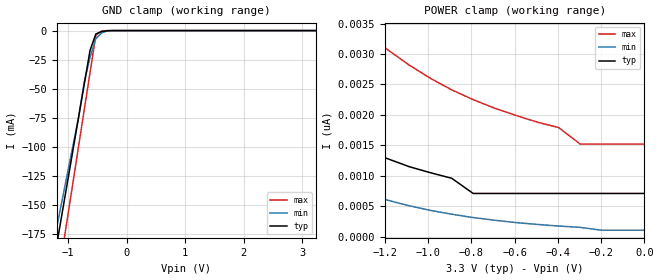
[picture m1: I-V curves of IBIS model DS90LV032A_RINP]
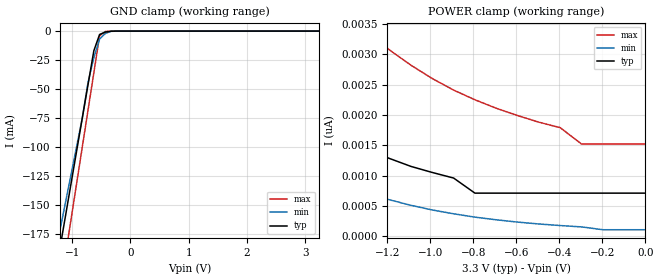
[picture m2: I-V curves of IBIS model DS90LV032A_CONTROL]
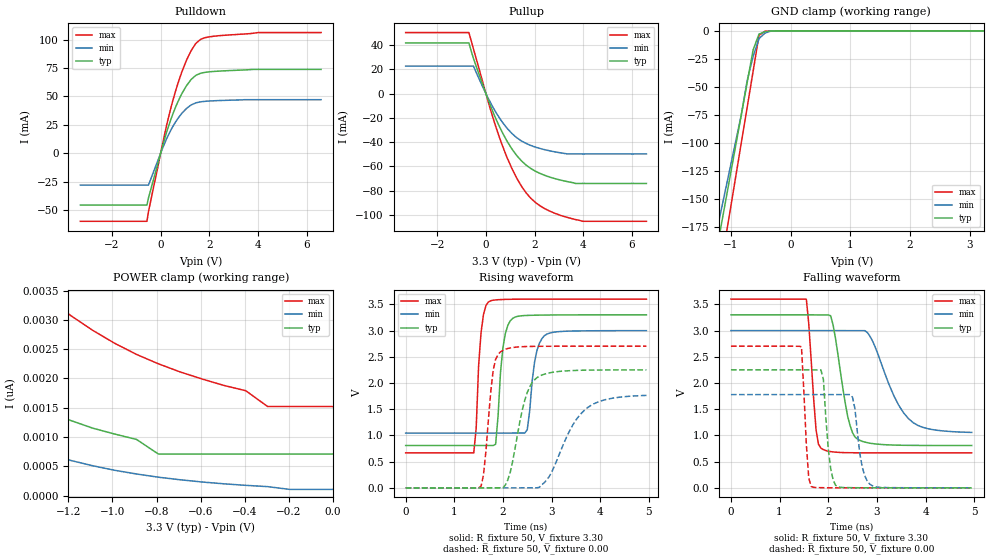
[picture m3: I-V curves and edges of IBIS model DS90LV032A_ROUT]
|   National Semiconductor Corporation
|   IBIS Model of DS90LV032A
|   3V LVDS Quad CMOS Differential Line Receiver
|   16 Lead SOIC Package
[IBIS Ver]   3.2
[Comment Char]   |_char
[File name]   ds90lv032atm.ibs
[File Rev]   2.2
[Date]   01/21/04
[Source]   SPICE to IBIS Translation
[Notes]
IBIS Parser Results:
Checking ds90lv032atm.ibs for IBIS 3.2 Compatibility...
Errors  : 0
File Passed
* Rev 2.2 Comments:
- Revision date: 01/21/04
Model Comments:
- Corrected [Difff Pin] assignments for pin 14 and 15
- Modifed [Diff Pin} comments
Modified By: DG
* END Rev 2.2 Comments
* Rev 2.1 Comments:
- Revision date: 06/03/03
Model Comments:
- Updated package parasitics data- added min/max
- Modifed fall and rise waveforms so that they are monotonic
- Corrected gnd clamp and power clamp data
Modified By: DG
* END Rev 2.1 Comments
* Rev 1.1 Comments:
- Revision date: 03/20/03
Model Comments:
- This file includes typ/min/max data
- SPICE files used were from an equivalent I/O design cell
- The CONTROL Model represents the following pins: EN, ENb
Created By: Tim Coyle
* END Rev 1.1 Comments
[Disclaimer]
(C) Copyright National Semiconductor Corporation 2003
   All rights reserved
   National Semiconductor Corporation hereby grants
the user of this IBIS model a non-exclusive, nontransferable
license to use this IBIS model under the following terms.
Before using this IBIS model, the user should read this
license.  If the user does not accept these terms,  the
IBIS model should be returned to National within 30 days.
   The user is granted this license only to use the
IBIS model and is not granted rights to sell, load, rent,
lease or license the IBIS model in whole or in part, or in
modified form to anyone other than user. User may modify
the IBIS model to suit its specific applications but rights
to derivative works and such modifications shall belong to
National.
   This IBIS model is provided on an "AS IS" basis and
National makes absolutely no warranty with respect to the
information contained herein.NATIONAL DISCLAIMS AND CUSTOMER
WAIVES ALL WARRANTIES, EXPRESS OR IMPLIED, INCLUDING
WARRANTIES OF MERCHANTABILITY OR FITNESS FOR A PARTICULAR
PURPOSE. The entire risk as to quality and performance is
with the Customer. ACCORDINGLY, IN NO EVENT SHALL THE
COMPANY BE LIABLE FOR ANY DAMAGES, WHETHER IN CONTRACT OR
TORT,INCLUDING ANY LOST PROFITS OR OTHER INCIDENTAL,
CONSEQUENTIAL, EXEMPLARY, OR PUNITIVE DAMAGES ARISING OUT
OF THE USE OR APPLICATION OF THE IBIS model provided in
this package.Further, National reserves the right to make
changes without notice to any product herein to improve
reliability, function, or design. National does not convey
any license under patent rights or any other intellectual
property rights, including those of third parties.
   National is not obligated to provide maintenance or support
for the licensed IBIS model.
Contact National at
   ATTN:INTERFACE APPLICATIONS/IBIS MODELS
   5 Foden Road, M/S 03-03
   South Porltand, ME 04106
   (207) 541-6031
[Copyright]   (c) Copyright 2003 National Semiconductor Corp.
[Component]   DS90LV032ATM
Si_location Pin
Timing_location Pin
[Manufacturer]   National Semiconductor Corp.
[Package]
|   TYP   MIN   MAX
R_pkg   50.0m   50.0m   50.0m
L_pkg   1.37nH  0.95n   2.07n
C_pkg   0.26pF  0.146p  0.429p
[Pin]   signal_name   model_name   R_pin   L_pin   C_pin
1   Rin1-   DS90LV032A_RINM   50.0m   2.07n   0.429p
2   Rin1+   DS90LV032A_RINP   50.0m   1.49n   0.306p
3   Rout1   DS90LV032A_ROUT   50.0m   0.95n   0.146p
4   EN   DS90LV032A_CONTROL 50.0m   0.95n   0.152p
5   Rout2   DS90LV032A_ROUT   50.0m   0.95n   0.152p
6   Rin2+   DS90LV032A_RINP   50.0m   0.95n   0.146p
7   Rin2-   DS90LV032A_RINM   50.0m   1.49n   0.306p
8   GND   GND   50.0m   2.07n   0.429p
9   Rin3-   DS90LV032A_RINM   50.0m   2.07n   0.429p
10   Rin3+   DS90LV032A_RINP   50.0m   1.49n   0.306p
11   Rout3   DS90LV032A_ROUT   50.0m   0.95n   0.146p
12   EN*   DS90LV032A_CONTROL 50.0m   0.95n   0.152p
13   Rout4   DS90LV032A_ROUT   50.0m   0.95n   0.152p
14   Rin4+   DS90LV032A_RINP   50.0m   0.95n   0.146p
15   Rin4-   DS90LV032A_RINM   50.0m   1.49n   0.306p
16   Vcc   POWER   50.0m   2.07n   0.429p
[Diff Pin] inv_pin   vdiff   tdelay_typ   tdelay_min   tdelay_max
| The '+' pin is Diff_pin and the '-' pin is the inv_pin
| Vdiff for Inputs is differential threshold Vth/Vtl (from datasheet)
| Vdiff is 0 for Outputs
| The 'tdelay' parameters are for specifying launch delays of the
| non-inverting pin relative to the inverting pin
| The 'tdelay' for Inputs is NA;  For LVDS Outputs it is 0ns since there
| is no transistor delay between the diff. pairs;
| the package delay is reflected by the  L_pin in the [Pin] keyword.
2   1   100mV   NA   NA   NA
6   7   100mV   NA   NA   NA
10   9   100mV   NA   NA   NA
14   15   100mV   NA   NA   NA
| Models and submodels in the file (4): DS90LV032A_RINP (Input), DS90LV032A_RINM (Input), DS90LV032A_CONTROL (Input), DS90LV032A_ROUT (3-state)
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[Model]   DS90LV032A_RINP
Model_type Input
Vinh=0.1
Vinl=-0.1
|   TYP   MIN   MAX
C_comp   2.25p   1p   2.75p
[Temperature Range] 25   85   -40
[Voltage Range]   3.30   3.00   3.60
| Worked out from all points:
|   GND clamp passes 1 mA (typ) near -0.44 V on its own axis
[GND Clamp]
|V(groundclamp)   I(typ)   I(min)   I(max)
-3.3V     -800mA     -700mA     -900mA
-1.221V   -191mA     -175mA     -228mA
-1.122V   -162mA     -150mA     -196mA
-1.023V   -133mA     -125mA     -164mA
-825mV    -75mA      -75mA      -100mA
-726mV    -46mA      -44.2mA    -68mA
-627mV    -17mA      -22.9mA    -36mA
-528mV    -2.88mA    -6.91mA    -4mA
-429mV    -868uA     -2.06mA    -342uA
-330mV    -103uA     -230uA     -43.7uA
-231mV    -7.76uA    -11.5uA    -4.83uA
3.234V    245pA      53.3pA     1.12nA
[POWER Clamp]
|V(table)   I(typ)   I(min)   I(max)
-3.267V   19.9nA     16nA       32nA
-2.277V   5.16nA     3.62nA     10.2nA
-2.178V   4.5nA      3.09nA     9.04nA
-1.98V    3.42nA     2.24nA     7.15nA
-1.683V   2.29nA     1.37nA     5.09nA
-1.287V   1.42nA     707pA      3.37nA
-1.089V   1.15nA     508pA      2.82nA
-891mV    958pA      368pA      2.41nA
-792mV    709pA      313pA      2.25nA
-396mV    709pA      174pA      1.79nA
-297mV    709pA      152pA      1.52nA
0V        709pA      105pA      1.52nA
[Model]   DS90LV032A_CONTROL
Model_type Input
Vinh=2.0
Vinl=0.8
|   TYP   MIN   MAX
C_comp   3p   3p   3p
[Temperature Range] 25   85   -40
[Voltage Range]   3.30   3.00   3.60
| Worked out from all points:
|   GND clamp passes 1 mA (typ) near -0.44 V on its own axis
[GND Clamp]
|V(groundclamp)   I(typ)   I(min)   I(max)
-3.3V     -800mA     -700mA     -900mA
-1.221V   -191mA     -175mA     -228mA
-1.122V   -162mA     -150mA     -196mA
-1.023V   -133mA     -125mA     -164mA
-825mV    -75mA      -75mA      -100mA
-726mV    -46mA      -44.2mA    -68mA
-627mV    -17mA      -22.9mA    -36mA
-528mV    -2.88mA    -6.91mA    -4mA
-429mV    -868uA     -2.06mA    -342uA
-330mV    -103uA     -230uA     -43.7uA
-231mV    -7.76uA    -11.5uA    -4.83uA
3.234V    245pA      53.3pA     1.12nA
[POWER Clamp]
|V(table)   I(typ)   I(min)   I(max)
-3.267V   19.9nA     16nA       32nA
-2.277V   5.16nA     3.62nA     10.2nA
-2.178V   4.5nA      3.09nA     9.04nA
-1.98V    3.42nA     2.24nA     7.15nA
-1.683V   2.29nA     1.37nA     5.09nA
-1.287V   1.42nA     707pA      3.37nA
-1.089V   1.15nA     508pA      2.82nA
-891mV    958pA      368pA      2.41nA
-792mV    709pA      313pA      2.25nA
-396mV    709pA      174pA      1.79nA
-297mV    709pA      152pA      1.52nA
0V        709pA      105pA      1.52nA
[Model]   DS90LV032A_ROUT
Model_type 3-state
Enable Active-High
Polarity Non-Inverting
Vref=0.0
Vmeas=1.65
Cref=10p
|   TYP   MIN   MAX
C_comp   4.2p   3.7p   4.9p
[Temperature Range] 25   85   -40
[Voltage Range]   3.30   3.00   3.60
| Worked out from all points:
|   slope of the pulldown table from 0 to 0.495 V, typ, clamps not added: 14.5 ohm
|   slope of the pullup table from 0 to 0.495 V, typ, clamps not added: 20.2 ohm
|   GND clamp passes 1 mA (typ) near -0.44 V on its own axis
|   falling waveform, R_fixture 50, V_fixture 3.30: 20-80 % time 258ps typ, 543ps min, 129ps max; typ from 3.3 V to 0.808 V
|   falling waveform, R_fixture 50, V_fixture 0.00: 20-80 % time 121ps typ, 153ps min, 92ps max; typ from 2.25 V to 0 V
|   rising waveform, R_fixture 50, V_fixture 3.30: 20-80 % time 130ps typ, 151ps min, 103ps max; typ from 0.808 V to 3.3 V
|   rising waveform, R_fixture 50, V_fixture 0.00: 20-80 % time 307ps typ, 572ps min, 157ps max; typ from 0 V to 2.25 V
[Pullup]
|Vtable   I(typ)   I(min)   I(max)
-3.3V     41.78mA    22.7mA     50.33mA
-700mV    41.78mA    22.7mA     50.33mA
-512mV    29.03mA    22.7mA     36.91mA
300mV     -15.55mA   -11.59mA   -20.51mA
862mV     -38.95mA   -28.35mA   -52.32mA
1.425V    -54.59mA   -38.51mA   -75.06mA
1.675V    -59.21mA   -41.24mA   -82.3mA
2.05V     -64.06mA   -44.15mA   -89.91mA
2.862V    -70.17mA   -48.06mA   -98.81mA
3.675V    -73.99mA   -49.71mA   -103.7mA
3.987V    -73.99mA   -49.71mA   -105.2mA
6.6V      -73.99mA   -49.71mA   -105.2mA
[Pulldown]
|V(pulldown)   I(typ)   I(min)   I(max)
-3.3V     -45.6mA    -28.09mA   -59.93mA
-562.5mV  -45.6mA    -28.09mA   -59.93mA
-500mV    -39.41mA   -28.09mA   -51.57mA
250mV     18.81mA    12.97mA    24.97mA
625mV     41.14mA    27.9mA     55.5mA
875mV     52.59mA    35.22mA    71.76mA
1.062V    59.45mA    39.4mA     81.87mA
1.438V    68.45mA    44.3mA     96.41mA
1.625V    70.29mA    45.22mA    99.98mA
2.188V    72.04mA    46.22mA    103.1mA
4V        73.87mA    47.18mA    106.3mA
6.6V      73.87mA    47.18mA    106.3mA
[GND Clamp]
|V(groundclamp)   I(typ)   I(min)   I(max)
-3.3V     -800mA     -700mA     -900mA
-1.221V   -191mA     -175mA     -228mA
-1.122V   -162mA     -150mA     -196mA
-1.023V   -133mA     -125mA     -164mA
-825mV    -75mA      -75mA      -100mA
-726mV    -46mA      -44.2mA    -68mA
-627mV    -17mA      -22.9mA    -36mA
-528mV    -2.88mA    -6.91mA    -4mA
-429mV    -868uA     -2.06mA    -342uA
-330mV    -103uA     -230uA     -43.7uA
-231mV    -7.76uA    -11.5uA    -4.83uA
3.234V    245pA      53.3pA     1.12nA
[POWER Clamp]
|V(table)   I(typ)   I(min)   I(max)
-3.267V   19.9nA     16nA       32nA
-2.277V   5.16nA     3.62nA     10.2nA
-2.178V   4.5nA      3.09nA     9.04nA
-1.98V    3.42nA     2.24nA     7.15nA
-1.683V   2.29nA     1.37nA     5.09nA
-1.287V   1.42nA     707pA      3.37nA
-1.089V   1.15nA     508pA      2.82nA
-891mV    958pA      368pA      2.41nA
-792mV    709pA      313pA      2.25nA
-396mV    709pA      174pA      1.79nA
-297mV    709pA      152pA      1.52nA
0V        709pA      105pA      1.52nA
[Ramp]
|   TYP   MIN   MAX
dV/dt_r   1.496V/0.258ns   1.160V/0.540ns   1.758V/0.127ns
dV/dt_f   1.349V/0.305ns   1.059V/0.586ns   1.620V/0.152ns
R_load=50
[Falling Waveform]
R_fixture=50
V_fixture=3.30
V_fixture_min=3.00
V_fixture_max=3.60
|Time   V(typ)   V(min)   V(max)
0s        3.3V       3V         3.6V
1.55ns    3.3V       3V         3.599V
1.75ns    3.299V     3V         1.105V
1.85ns    3.298V     3V         757mV
2.05ns    3.283V     3V         691mV
2.4ns     1.363V     2.999V     671mV
2.55ns    971mV      2.999V     669mV
2.85ns    853mV      2.905V     668mV
3.65ns    811mV      1.32V      668mV
4.95ns    808mV      1.057V     668mV
[Falling Waveform]
R_fixture=50
V_fixture=0.00
V_fixture_min=0.00
V_fixture_max=0.00
|Time   V(typ)   V(min)   V(max)
0s        2.251V     1.779V     2.702V
1.45ns    2.251V     1.779V     2.692V
1.55ns    2.251V     1.779V     831mV
1.65ns    2.251V     1.779V     26.9mV
1.9ns     2.071V     1.779V     2.86mV
2ns       746mV      1.779V     1.7mV
2.15ns    50.1mV     1.779V     783uV
2.5ns     3.28mV     1.728V     174uV
2.9ns     911uV      43.5mV     55.1uV
4.95ns    21.7uV     183uV      1.59uV
[Rising Waveform]
R_fixture=50
V_fixture=3.30
V_fixture_min=3.00
V_fixture_max=3.60
|Time   V(typ)   V(min)   V(max)
0s        808mV      1.045V     668mV
1.4ns     808mV      1.045V     668mV
1.55ns    808mV      1.045V     2.96V
1.7ns     808mV      1.045V     3.544V
1.85ns    832mV      1.045V     3.585V
2ns       2.675V     1.045V     3.593V
2.2ns     3.232V     1.046V     3.598V
2.5ns     3.289V     1.108V     3.599V
2.85ns    3.296V     2.9V       3.6V
4.95ns    3.3V       2.999V     3.6V
[Rising Waveform]
R_fixture=50
V_fixture=0.00
V_fixture_min=0.00
V_fixture_max=0.00
|Time   V(typ)   V(min)   V(max)
0s        2.1nV      24.2nV     108pV
1.55ns    1.94uV     22.5nV     29mV
1.6ns     72.5nV     24.1nV     244mV
1.8ns     840uV      23.8nV     2.245V
2ns       840uV      717nV      2.623V
2.15ns    295mV      1.64uV     2.668V
2.45ns    1.674V     912uV      2.695V
2.7ns     2.102V     912uV      2.7V
3.7ns     2.245V     1.5V       2.702V
4.95ns    2.25V      1.763V     2.702V
